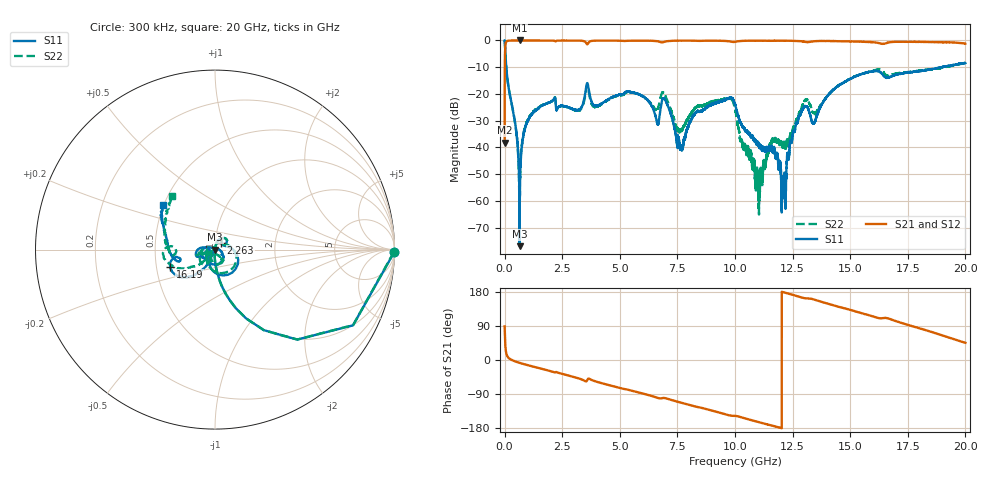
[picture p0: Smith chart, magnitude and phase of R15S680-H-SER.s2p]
!{R15S680}
!Johanson Technology Inc.
!www.johansontechnology.com
!Test Board Conditions:
!Substrate Type  RO4350B
!Substrate Thickness  20 mil
!Substrate Dk  3.66
!TL Type: GCPW
!TL Trace Width  34 mil
!TL Gap  10 mil
!Electrode orientation  Horizontal
!DUT TOPOLOGY	SERIES
!Mounting Pad LxW  26x52 mil
! Created Sat Feb  6 14:35:08 2021
# hz S ma R 50
! 2 Port Network Data from SP1.SP block
! freq  magS11  angS11  magS21  angS21  magS12  angS12  magS22  angS22
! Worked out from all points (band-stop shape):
!   20001 points, 300 kHz to 20 GHz, reference 50 ohm
!   highest |S21| = 0.00 dB at 648.3 MHz (marker M1); lowest = -38.2 dB at 300 kHz (marker M2)
!   |S21| within 3 dB of the highest: 24.49 MHz to end of sweep
!   lowest |S11| = -76.9 dB at 652.3 MHz (marker M3), VSWR 1.00, Z = 50 - j0.00965 ohm
!   |S11| at or under -10 dB: 72.22 MHz to 18.93 GHz (18.85 GHz wide, 198 % of centre)
!   |S22| runs from -70.5 to 0.0 dB; largest |S21 - S12| = 0.016
!   S11 on the Smith chart (normalised r, x): 300 kHz: open; 2.263 GHz: 1.07, +0.08; 16.19 GHz: 0.59, -0.12; 20 GHz: 0.50, +0.29
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300000  0.9978 -0.9  0.01234 88.8  0.01232 88.8  0.9964 -0.8
1.133e8  0.2049 -79.4  0.9781 10.4  0.978 10.4  0.2058 -79.4
6.483e8  0.0004855 -115.3  0.9999 -7.5  0.9985 -7.4  0.000298 160.7
6.523e8  0.0001428 -137.5  0.9994 -7.5  0.9995 -7.5  0.0009172 118.9
1.0973e9  0.03736 75.6  0.9985 -15.2  0.9984 -15.1  0.03855 75.9
2.2633e9  0.05001 46.8  0.9865 -32.1  0.9864 -32.1  0.05082 44.0
3.3343e9  0.05641 23.1  0.9892 -51.0  0.989 -50.9  0.05405 37.0
3.5863e9  0.1598 -51.0  0.8456 -53.0  0.8466 -52.9  0.1438 -51.5
5.4393e9  0.1089 -168.0  0.987 -79.8  0.9881 -79.8  0.1077 -167.5
6.6673e9  0.02757 -151.6  0.9625 -100.4  0.9628 -100.3  0.05539 -122.2
6.9593e9  0.07842 -169.9  0.9507 -100.5  0.9507 -100.4  0.09653 -151.8
7.6753e9  0.0103 75.1  0.9907 -112.9  0.9915 -112.9  0.02075 -95.5
8.3183e9  0.04589 -27.2  0.9854 -123.3  0.9846 -123.3  0.05671 -56.3
1.00003e10  0.0654 -123.3  0.9427 -147.4  0.9432 -147.4  0.05306 -116.2
1.09813e10  0.0123 -149.1  0.9902 -163.2  0.9876 -163.2  0.002884 30.0
1.15813e10  0.009702 139.8  0.9852 -172.8  0.9847 -172.7  0.01227 132.8
1.21123e10  0.001758 170.4  0.987 178.7  0.9878 178.6  0.01221 153.2
1.28353e10  0.04064 -123.8  0.971 166.0  0.9707 166.0  0.0475 -139.5
1.33343e10  0.03025 -164.8  0.9542 161.3  0.954 161.2  0.0497 178.5
1.61863e10  0.2672 -158.9  0.9038 111.2  0.9034 111.3  0.288 -170.1
1.66673e10  0.201 -162.7  0.9191 109.2  0.9072 109.2  0.2193 -175.8
2e10  0.3776 139.1  0.874 45.3  0.8655 45.1  0.3807 128.4
